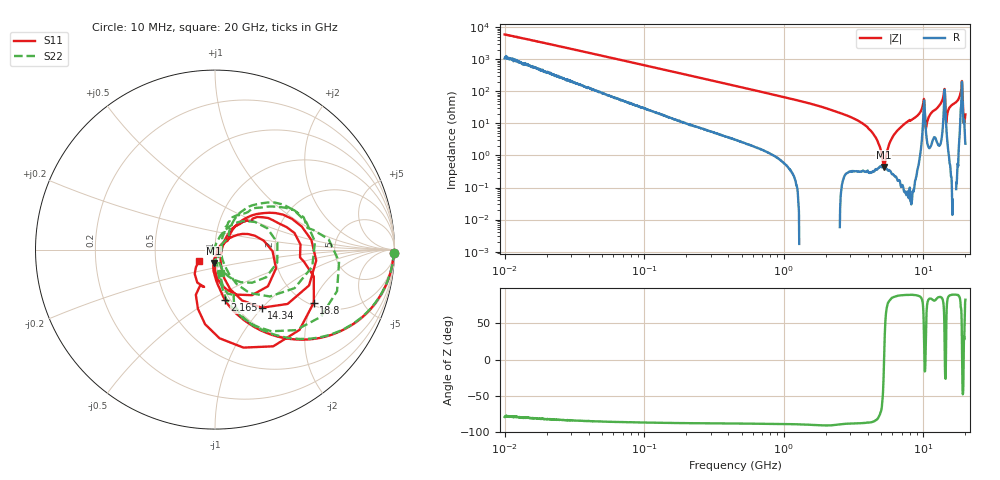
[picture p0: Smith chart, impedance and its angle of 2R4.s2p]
!Keysight Technologies,P5008B,MY61100088,A.16.20.02
!Date: Monday, October 30, 2023 16:28:18
!Correction: S11(C  2-Port  )
!S21(C  2-Port  )
!S12(C  2-Port  )
!S22(C  2-Port  )
!S2P File: Measurements: S11, S21, S12, S22:Log Frequency Sweep
# Hz S  dB  R 50
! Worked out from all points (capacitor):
!   1601 points, 10 MHz to 20 GHz, reference 50 ohm
!   read as one part in series: C = 2.64 pF near 10.39 MHz
!   lowest |Z| = 437 mohm at 5.214 GHz (marker M1)
!   series resonance near 5.229 GHz, so ESL is about 350 pH
!   S11 on the Smith chart (normalised r, x): 10 MHz: open; 2.165 GHz: 0.95, -0.58; 14.34 GHz: 1.27, -0.99; 18.8 GHz: 2.11, -2.04; 20 GHz: 0.83, -0.11
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1e7  -0.02 -1.0  -35.56 78.7  -35.57 78.7  -0.03 -1.0
3.555162e7  -0.05 -3.2  -25.15 81.9  -25.15 81.9  -0.05 -3.2
1.263918e8  -0.22 -11.0  -14.56 76.8  -14.57 76.8  -0.22 -10.9
4.472136e8  -1.68 -34.1  -5.20 54.9  -5.21 54.9  -1.68 -33.8
1.589917e9  -8.17 -70.5  -0.68 20.8  -0.69 20.8  -8.17 -69.4
2.165104e9  -10.86 -78.7  -0.32 13.4  -0.32 13.4  -10.96 -77.1
5.213871e9  -22.48 -95.8  -0.04 -4.2  -0.04 -4.2  -22.44 -82.8
5.652411e9  -24.17 -95.6  -0.03 -5.9  -0.03 -5.9  -24.18 -85.8
7.733948e9  -31.57 -11.7  0.01 -13.3  0.00 -13.4  -33.26 161.6
8.464494e9  -35.78 -25.2  0.01 -16.2  0.01 -16.2  -39.21 159.3
9.003717e9  -32.74 26.5  -0.00 -18.8  -0.01 -18.8  -33.64 84.7
9.995649e9  -11.17 10.3  -1.68 -32.1  -1.69 -32.2  -11.34 34.6
1.033363e10  -14.22 -80.3  -0.96 -10.2  -0.97 -10.2  -14.26 -59.0
1.078503e10  -27.03 -86.1  -0.15 -18.0  -0.15 -18.0  -26.33 -67.1
1.109686e10  -34.50 -11.7  -0.11 -20.6  -0.12 -20.7  -32.39 -6.4
1.298028e10  -14.38 48.5  -0.31 -30.4  -0.31 -30.5  -14.26 57.2
1.374174e10  -8.74 34.2  -1.09 -40.3  -1.09 -40.3  -8.79 45.1
1.434201e10  -7.62 -51.1  -3.51 -5.1  -3.52 -5.1  -7.91 -40.5
1.518335e10  -20.57 48.0  -0.11 -27.4  -0.12 -27.5  -19.90 60.7
1.767617e10  -11.55 38.2  -0.60 -47.9  -0.60 -47.9  -10.69 48.3
1.880222e10  -4.09 -28.2  -7.90 -63.3  -7.90 -63.3  -3.17 -5.5
2e10  -19.17 -144.3  -0.31 -28.7  -0.31 -28.8  -17.44 -76.1
